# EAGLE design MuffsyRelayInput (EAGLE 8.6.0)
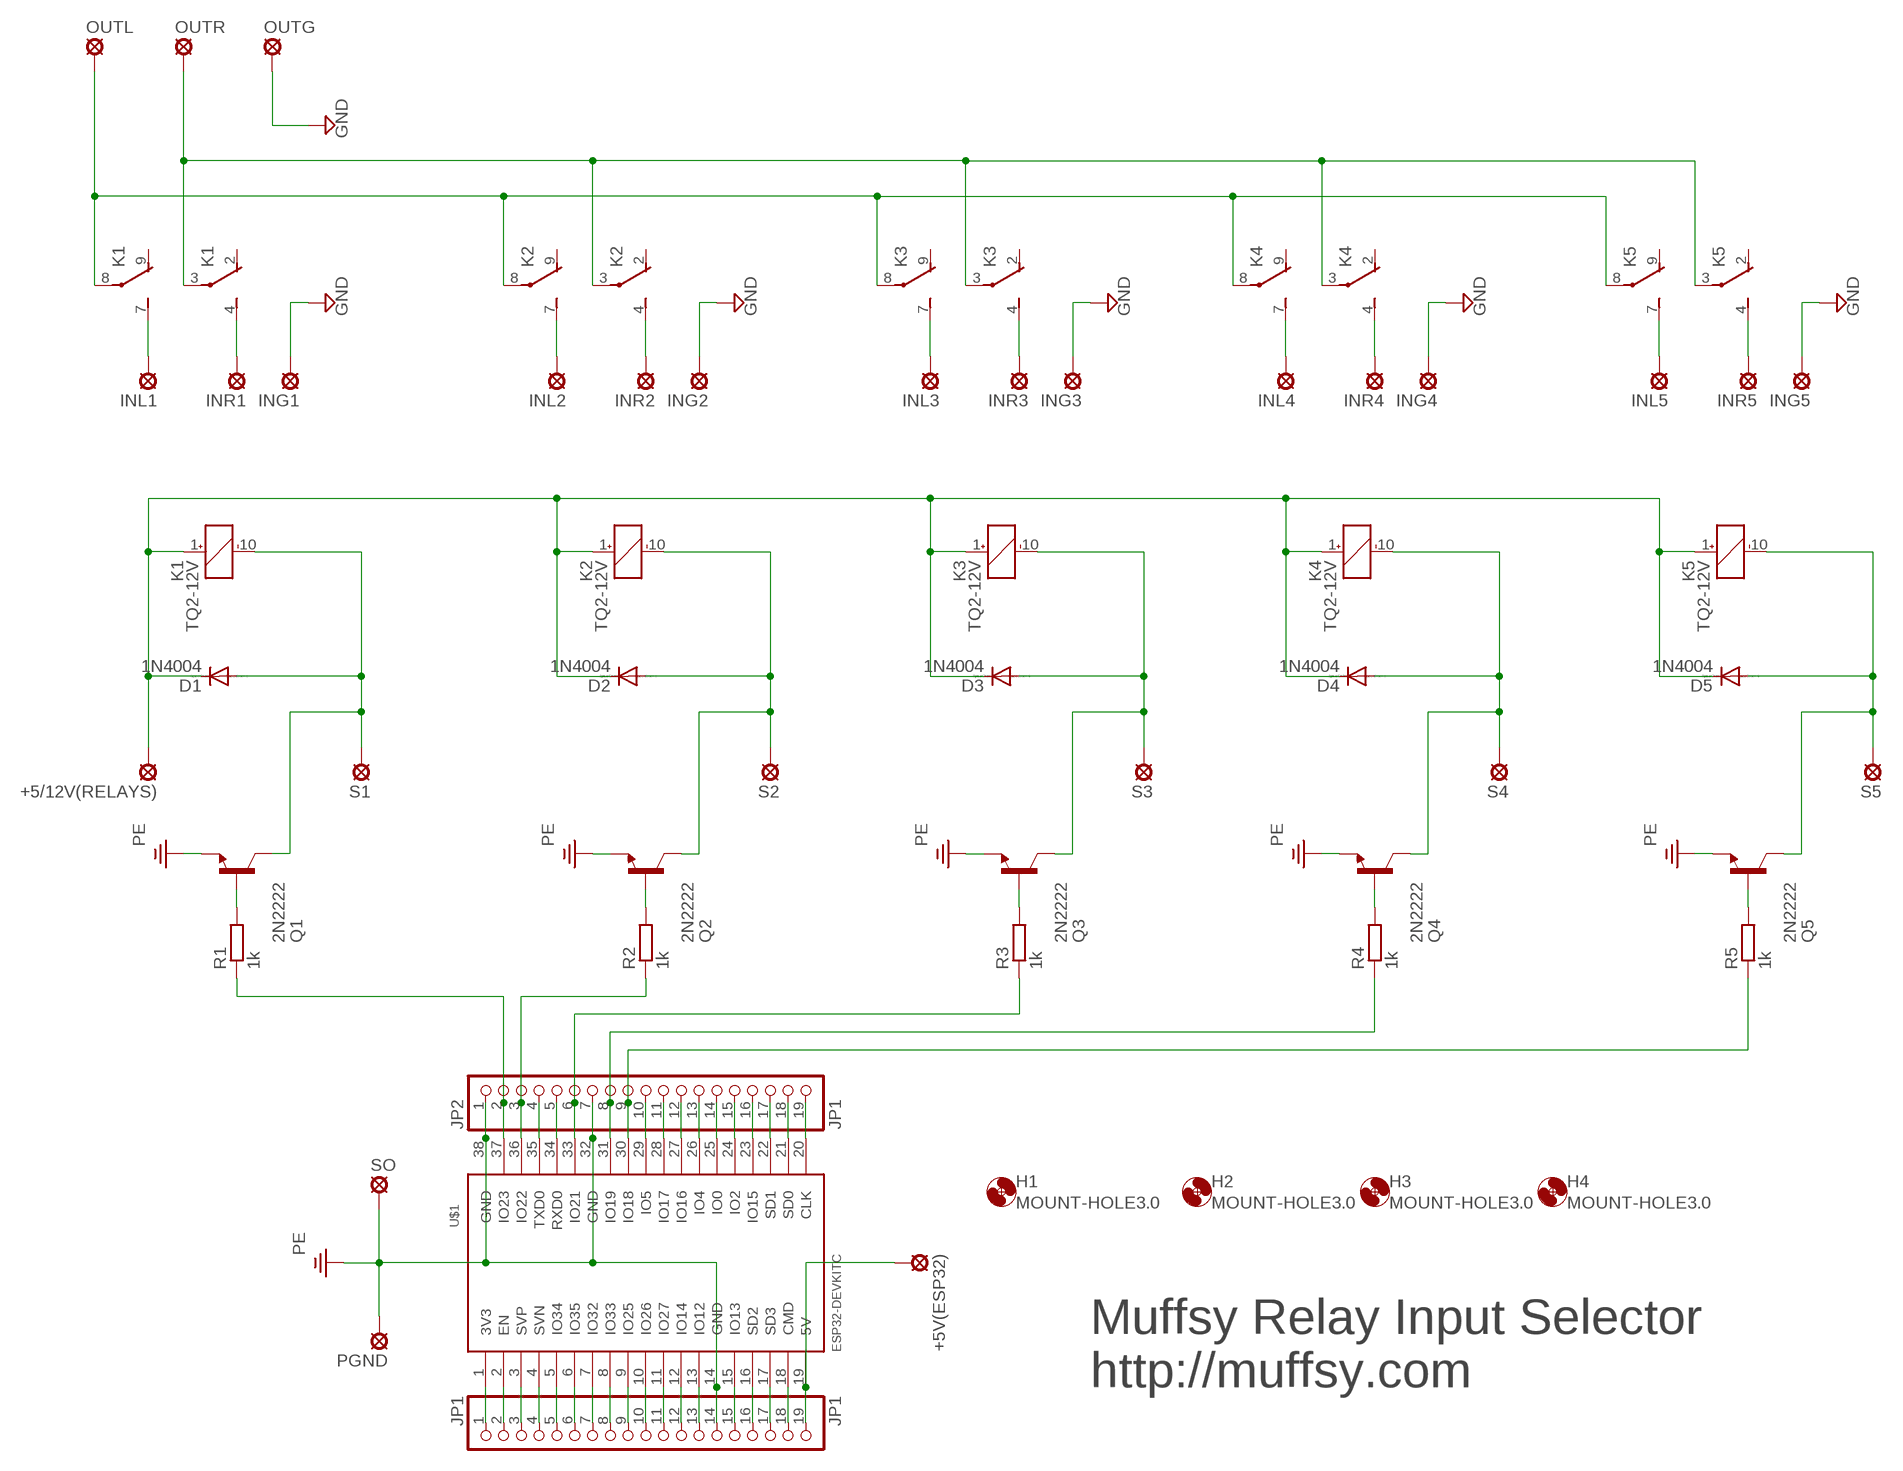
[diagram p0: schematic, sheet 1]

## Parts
+5/12V(RELAYS)  SE11  [SE11]
+5V(ESP32)  SE11  [SE11]
D1  1N4004  [DO41-10]
D2  1N4004  [DO41-10]
D3  1N4004  [DO41-10]
D4  1N4004  [DO41-10]
D5  1N4004  [DO41-10]
H1  MOUNT-HOLE3.0  [3,0]
H2  MOUNT-HOLE3.0  [3,0]
H3  MOUNT-HOLE3.0  [3,0]
H4  MOUNT-HOLE3.0  [3,0]
ING1  SE11  [SE11]
ING2  SE11  [SE11]
ING3  SE11  [SE11]
ING4  SE11  [SE11]
ING5  SE11  [SE11]
INL1  SE11  [SE11]
INL2  SE11  [SE11]
INL3  SE11  [SE11]
INL4  SE11  [SE11]
INL5  SE11  [SE11]
INR1  SE11  [SE11]
INR2  SE11  [SE11]
INR3  SE11  [SE11]
INR4  SE11  [SE11]
INR5  SE11  [SE11]
JP1  JP1  PINHD-1X19  [1X19]
JP2  JP1  PINHD-1X19  [1X19]
K1  TQ2-12V  [TQ2]
K2  TQ2-12V  [TQ2]
K3  TQ2-12V  [TQ2]
K4  TQ2-12V  [TQ2]
K5  TQ2-12V  [TQ2]
OUTG  SE11  [SE11]
OUTL  SE11  [SE11]
OUTR  SE11  [SE11]
PGND  SE11  [SE11]
Q1  2N2222  [TO18]
Q2  2N2222  [TO18]
Q3  2N2222  [TO18]
Q4  2N2222  [TO18]
Q5  2N2222  [TO18]
R1  1k  R-EU_0207/10  [0207/10]
R2  1k  R-EU_0207/10  [0207/10]
R3  1k  R-EU_0207/10  [0207/10]
R4  1k  R-EU_0207/10  [0207/10]
R5  1k  R-EU_0207/10  [0207/10]
S1  SE11  [SE11]
S2  SE11  [SE11]
S3  SE11  [SE11]
S4  SE11  [SE11]
S5  SE11  [SE11]
SO  SE11  [SE11]
U$1  ESP32DEVKITC  [ESP32-DEVKITC]

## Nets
GND: ING1.MP ING2.MP ING3.MP ING4.MP ING5.MP OUTG.MP
N$1: INL2.MP K2.7(2:S)
N$2: INL1.MP K1.7(2:S)
N$3: INR1.MP K1.4(1:S)
N$4: INR2.MP K2.4(1:S)
N$5: INL3.MP K3.7(2:S)
N$6: INR3.MP K3.4(1:S)
N$7: INL4.MP K4.7(2:S)
N$8: INR4.MP K4.4(1:S)
N$9: INL5.MP K5.7(2:S)
N$10: INR5.MP K5.4(1:S)
N$11: Q1.2(B) R1.2
N$12: K1.3(1:P) K2.3(1:P) K3.3(1:P) K4.3(1:P) K5.3(1:P) OUTR.MP
N$13: K1.8(2:P) K2.8(2:P) K3.8(2:P) K4.8(2:P) K5.8(2:P) OUTL.MP
N$14: Q2.2(B) R2.2
N$15: +5/12V(RELAYS).MP D1.C D2.C D3.C D4.C D5.C K1.1(_:+) K2.1(_:+) K3.1(_:+) K4.1(_:+) K5.1(_:+)
N$16: Q3.2(B) R3.2
N$17: Q4.2(B) R4.2
N$18: Q5.2(B) R5.2
N$19: JP1.1 U$1.1(3V3)
N$20: D1.A K1.10(_:-) Q1.3(C) S1.MP
N$21: D2.A K2.10(_:-) Q2.3(C) S2.MP
N$22: D3.A K3.10(_:-) Q3.3(C) S3.MP
N$23: D4.A K4.10(_:-) Q4.3(C) S4.MP
N$24: D5.A K5.10(_:-) Q5.3(C) S5.MP
N$25: JP1.2 U$1.2(EN)
N$26: JP1.3 U$1.3(SVP)
N$27: JP1.4 U$1.4(SVN)
N$28: JP1.5 U$1.5(IO34)
N$29: JP1.6 U$1.6(IO35)
N$30: JP1.7 U$1.7(IO32)
N$31: JP1.8 U$1.8(IO33)
N$32: JP1.9 U$1.9(IO25)
N$33: JP1.10 U$1.10(IO26)
N$34: JP1.11 U$1.11(IO27)
N$35: JP1.12 U$1.12(IO14)
N$36: JP1.13 U$1.13(IO12)
N$38: JP1.15 U$1.15(IO13)
N$44: JP1.16 U$1.16(SD2)
N$45: JP1.17 U$1.17(SD3)
N$46: JP1.18 U$1.18(CMD)
N$47: +5V(ESP32).MP JP1.19 U$1.19(5V)
N$49: JP2.2 R1.1 U$1.37(IO23)
N$50: JP2.3 R2.1 U$1.36(IO22)
N$51: JP2.4 U$1.35(TXD0)
N$52: JP2.5 U$1.34(RXD0)
N$53: JP2.6 R3.1 U$1.33(IO21)
N$55: JP2.8 R4.1 U$1.31(IO19)
N$56: JP2.9 R5.1 U$1.30(IO18)
N$57: JP2.10 U$1.29(IO5)
N$58: JP2.11 U$1.28(IO17)
N$59: JP2.12 U$1.27(IO16)
N$60: JP2.13 U$1.26(IO4)
N$61: JP2.14 U$1.25(IO0)
N$62: JP2.15 U$1.24(IO2)
N$63: JP2.16 U$1.23(IO15)
N$64: JP2.17 U$1.22(SD1)
N$65: JP2.18 U$1.21(SD0)
N$66: JP2.19 U$1.20(CLK)
PE: JP1.14 JP2.1 JP2.7 PGND.MP Q1.1(E) Q2.1(E) Q3.1(E) Q4.1(E) Q5.1(E) SO.MP U$1.14(GND) U$1.32(GND) U$1.38(GND)
Unconnected: K1.2(1:O) K1.9(2:O) K2.2(1:O) K2.9(2:O) K3.2(1:O) K3.9(2:O) K4.2(1:O) K4.9(2:O) K5.2(1:O) K5.9(2:O)

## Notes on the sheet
- Muffsy Relay Input Selector
- http://muffsy.com

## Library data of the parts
+5/12V(RELAYS) +5V(ESP32) ING1-ING5 INL1-INL5 INR1-INR5 OUTG OUTL OUTR PGND S1-S5 SO = relswitch:SE11: SOLDER PAD
D1-D5 = relswitch:1N4004: DIODE
H1-H4 = relswitch:MOUNT-HOLE: MOUNTING HOLE with drill center marker
JP1 JP2 = relswitch:PINHD-1X19: PIN HEADER
K1-K5 = relswitch:TQ2?*: LOW PROFILE 2 FORM C RELAY NAiS Source: http://www.mew-europe.com/.. en_ds_61020_0001.pdf Source: http://www.mew-europe.com/.. en_ds_61020_0004.pdf; MF: AROMAT/ MATSUSHITA; MPN: TQ2-12V; OC_FARNELL: 1200949; OC_NEWARK: 64K3197
Q1-Q5 = relswitch:2N2222*: NPN Transistor
R1-R5 = relswitch:R-EU_: RESISTOR, European symbol
U$1 = relswitch:ESP32DEVKITC

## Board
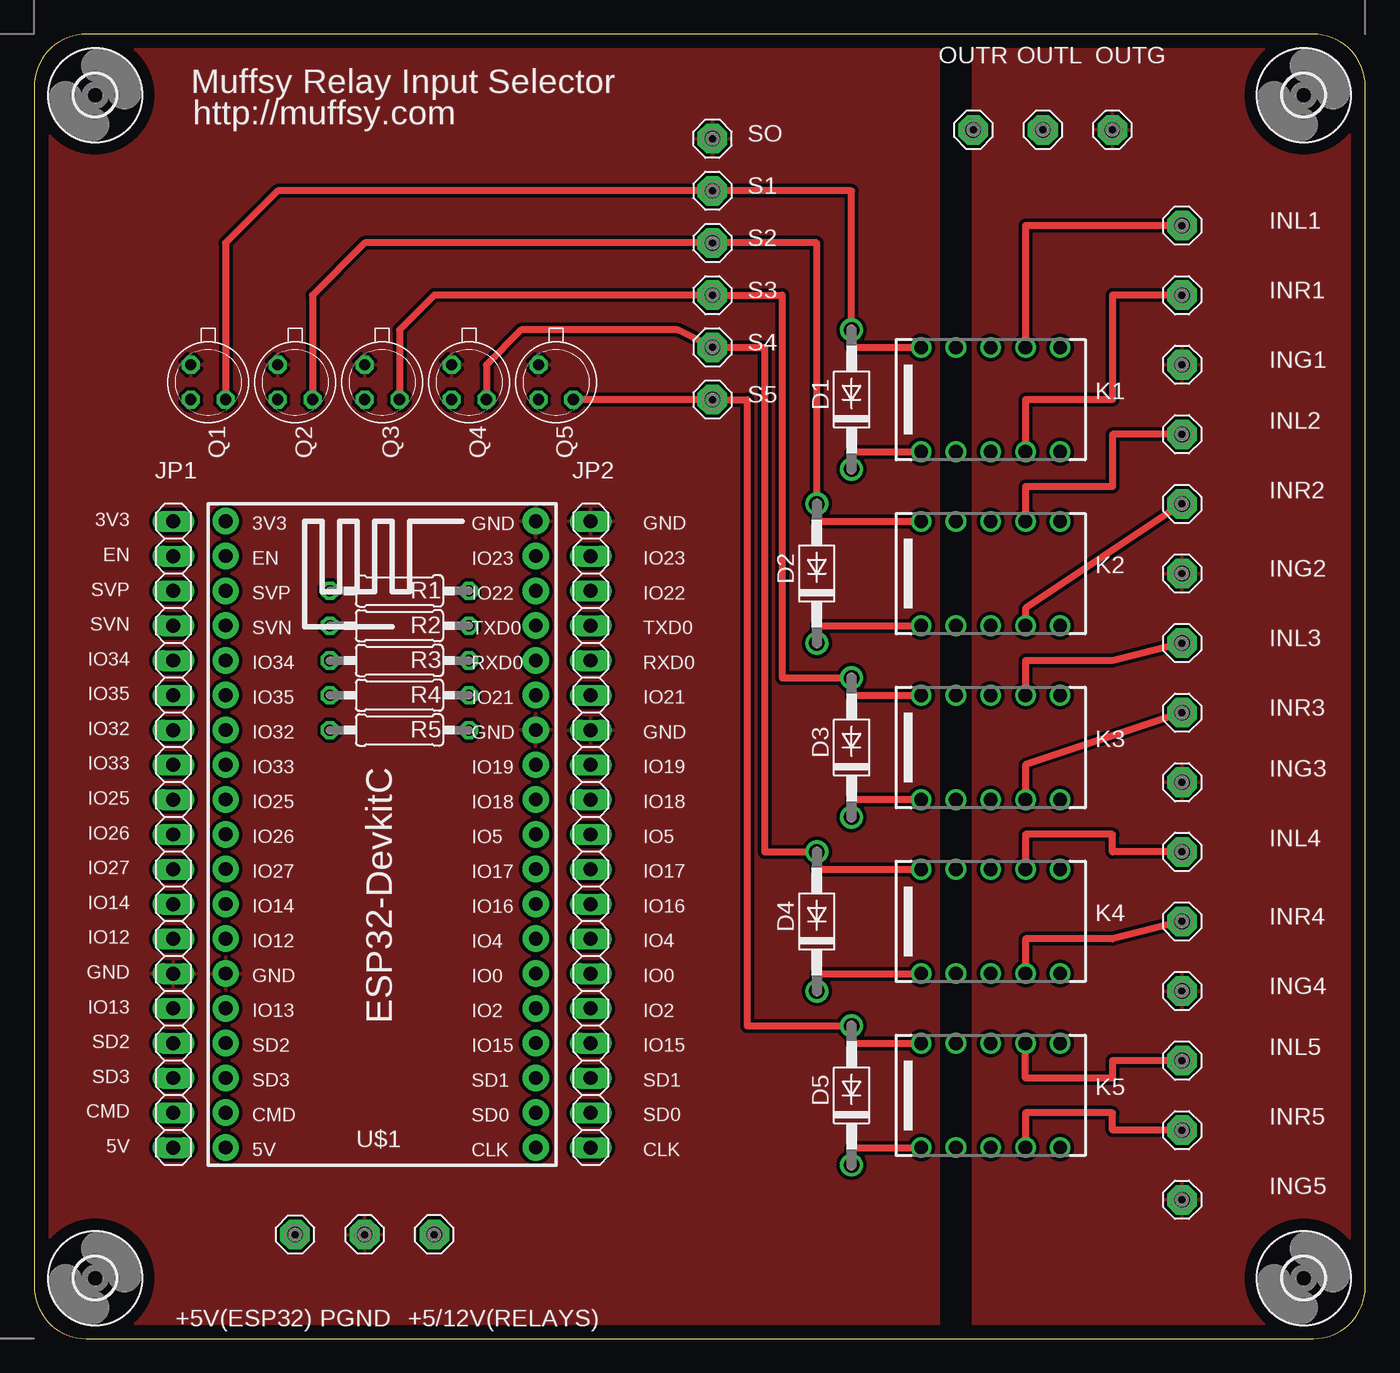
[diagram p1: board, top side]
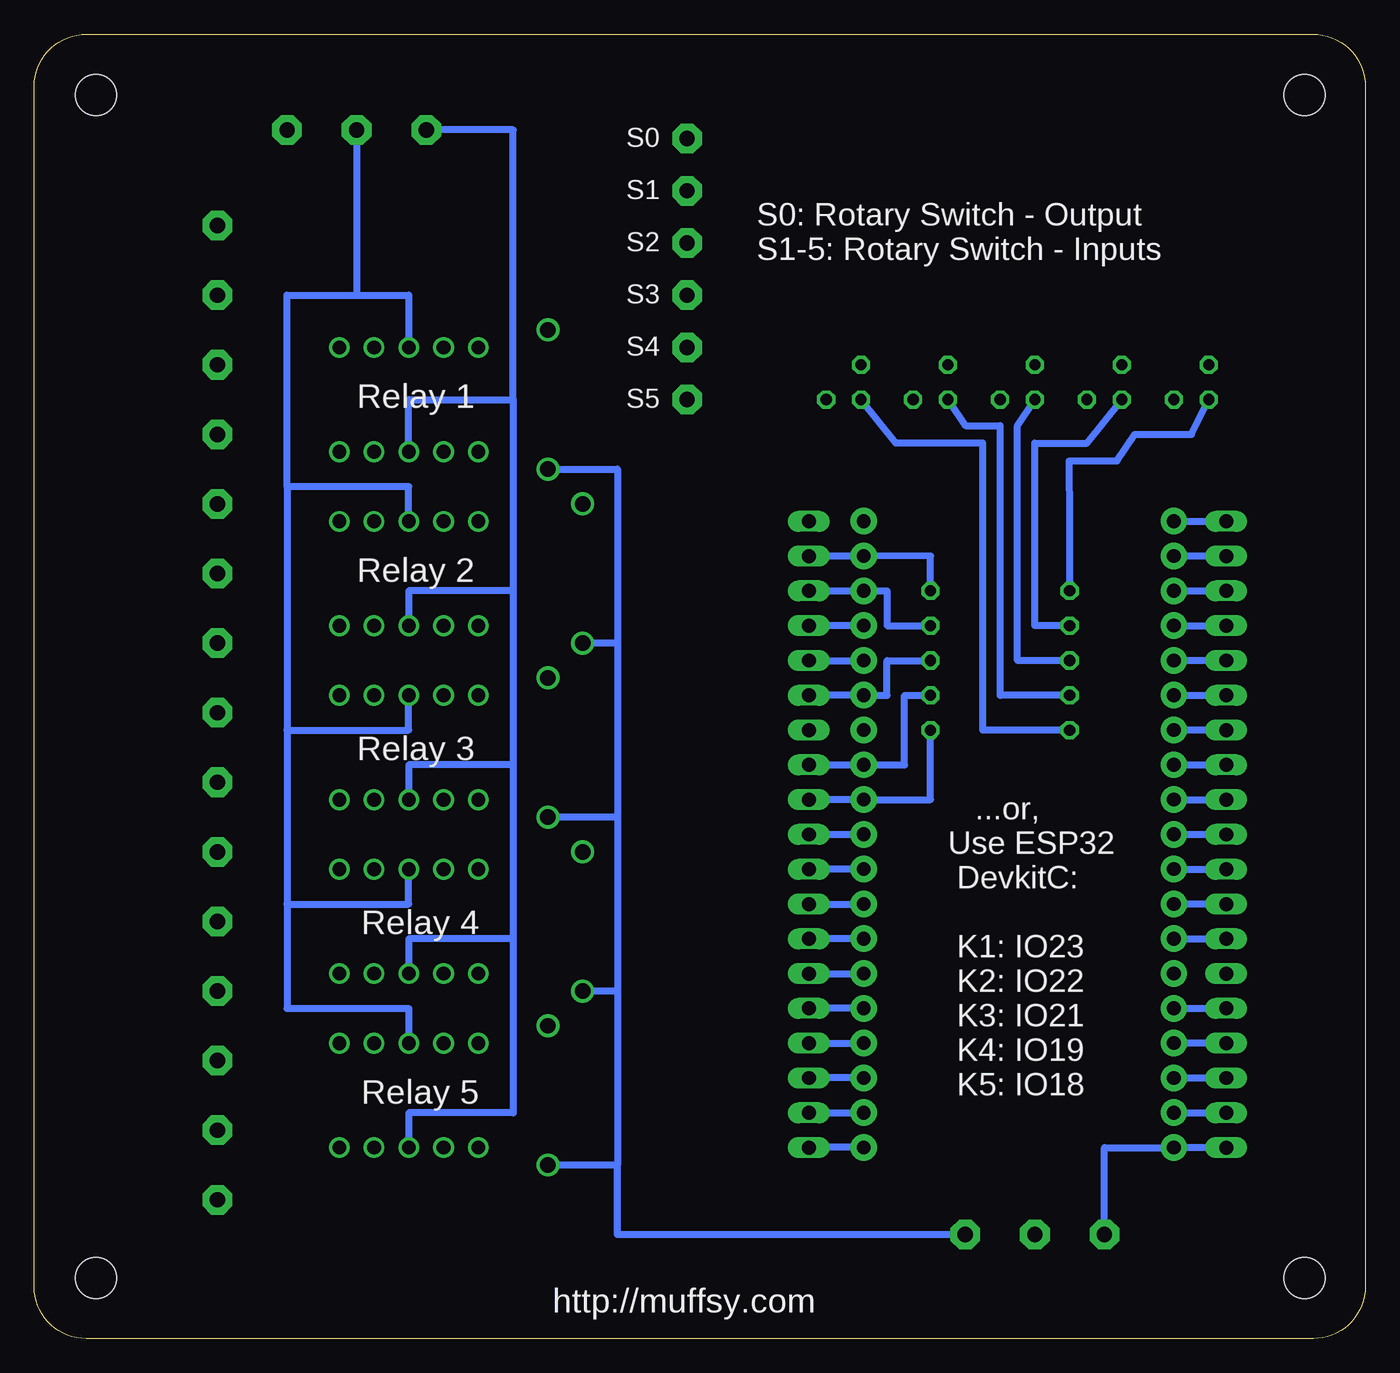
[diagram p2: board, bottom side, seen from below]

Size 97.21 x 95.23 mm. Coordinates in mm from the lower left corner, seen from the top.
Outline: 97.21,3.79 97.21,91.42 arc90 93.4,95.23 3.81,95.23 arc90 0,91.42 0,3.81 arc90 3.81,0 93.42,0 arc90 97.21,3.79
Copper layers (1*16): Top 0.035mm / dielectric 1.5mm / Bottom 0.035mm
Design rules "default": minimum track width 6mil, minimum drill 0.35mm, track to track 6mil, track to pad 6mil, pad to pad 6mil, via to via 6mil, smd to smd 6mil, copper to edge 40mil, drill to drill 6mil, minimum pad ring 10mil, minimum via ring 8mil, stop-mask expansion 4mil, vias tented up to drill 0mil, thermal gap 10mil

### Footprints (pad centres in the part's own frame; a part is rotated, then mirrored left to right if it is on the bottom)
SE11 = drill 1.118 pad 2.159 octagon: MP 0,0
DO41-10 = drill 1.118: A 5.08,0; C -5.08,0
3,0 = hole 3: 0,0
1X19 = drill 1.016 long: 1 -22.86,0; 2 -20.32,0; 3 -17.78,0; 4 -15.24,0; 5 -12.7,0; 6 -10.16,0; 7 -7.62,0; 8 -5.08,0; 9 -2.54,0; 10 0,0; 11 2.54,0; 12 5.08,0; 13 7.62,0; 14 10.16,0; 15 12.7,0; 16 15.24,0; 17 17.78,0; 18 20.32,0; 19 22.86,0
TQ2 = drill 1: 1 -5.08,-3.81; 2 -2.54,-3.81; 3 0,-3.81; 4 2.54,-3.81; 5 5.08,-3.81; 6 5.08,3.81; 7 2.54,3.81; 8 0,3.81; 9 -2.54,3.81; 10 -5.08,3.81
TO18 = drill 0.813 octagon: 1 -1.27,-1.27; 2 1.27,-1.27; 3 1.27,1.27
0207/10 = drill 0.813 octagon: 1 -5.08,0; 2 5.08,0
ESP32-DEVKITC = drill 1 pad 1.93: 1 -22.87,-11.42; 2 -20.33,-11.42; 3 -17.79,-11.42; 4 -15.25,-11.42; 5 -12.71,-11.42; 6 -10.17,-11.42; 7 -7.63,-11.42; 8 -5.09,-11.42; 9 -2.55,-11.42; 10 -0.01,-11.42; 11 2.53,-11.42; 12 5.07,-11.42; 13 7.61,-11.42; 14 10.15,-11.42; 15 12.69,-11.42; 16 15.23,-11.42; 17 17.77,-11.42; 18 20.31,-11.42; 19 22.85,-11.42; 20 22.85,11.23; 21 20.31,11.23; 22 17.77,11.23; 23 15.23,11.23; 24 12.69,11.23; 25 10.15,11.23; 26 7.61,11.23; 27 5.07,11.23; 28 2.53,11.23; 29 -0.01,11.23; 30 -2.55,11.23; 31 -5.09,11.23; 32 -7.63,11.23; 33 -10.17,11.23; 34 -12.71,11.23; 35 -15.25,11.23; 36 -17.79,11.23; 37 -20.33,11.23; 38 -22.87,11.23

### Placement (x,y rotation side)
+5/12V(RELAYS)  29.21,7.6 270 top
+5V(ESP32)  19.05,7.6 180 top
D1  59.69,68.56 90 top
D2  57.15,55.86 90 top
D3  59.69,43.16 90 top
D4  57.15,30.46 90 top
D5  59.69,17.76 90 top
H1  92.71,4.43 0 top
H2  4.45,4.43 0 top
H3  92.71,90.79 0 top
H4  4.45,90.79 0 top
ING1  83.82,71.1 0 top
ING2  83.82,55.86 0 top
ING3  83.82,40.62 0 top
ING4  83.82,25.38 0 top
ING5  83.82,10.14 0 top
INL1  83.82,81.26 0 top
INL2  83.82,66.02 0 top
INL3  83.82,50.78 0 top
INL4  83.82,35.54 0 top
INL5  83.82,20.3 0 top
INR1  83.82,76.18 0 top
INR2  83.82,60.94 0 top
INR3  83.82,45.7 0 top
INR4  83.82,30.46 0 top
INR5  83.82,15.22 0 top
JP1  10.16,36.81 270 top
JP2  40.64,36.81 270 top
K1  69.85,68.56 0 top
K2  69.85,55.86 0 top
K3  69.85,43.16 0 top
K4  69.85,30.46 0 top
K5  69.85,17.76 0 top
OUTG  78.74,88.25 270 top
OUTL  73.66,88.25 270 top
OUTR  68.58,88.25 270 top
PGND  24.13,7.6 270 top
Q1  12.7,69.83 270 top
Q2  19.05,69.83 270 top
Q3  25.4,69.83 270 top
Q4  31.75,69.83 270 top
Q5  38.1,69.83 270 top
R1  26.67,54.59 180 top
R2  26.67,52.05 180 top
R3  26.67,49.51 180 top
R4  26.67,46.97 180 top
R5  26.67,44.43 180 top
S1  49.53,83.8 0 top
S2  49.53,79.99 0 top
S3  49.53,76.18 0 top
S4  49.53,72.37 0 top
S5  49.53,68.56 0 top
SO  49.53,87.61 180 top
U$1  25.4,36.81 270 top

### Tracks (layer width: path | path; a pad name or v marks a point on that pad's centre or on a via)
GND
  pour Top (isolate 0.254): 97.16,-0.02 97.16,95.23 68.58,95.23 68.58,-0.02
N$1
  Top 0.508: K2.7 72.39,62.21 78.74,62.21 78.74,66.02 INL2.MP
N$2
  Top 0.508: INL1.MP 72.39,81.26 K1.7
N$3
  Top 0.508: INR1.MP 78.74,76.18 78.74,68.56 72.39,68.56 K1.4
N$4
  Top 0.508: INR2.MP 72.39,53.32 K2.4
N$5
  Top 0.508: INL3.MP 78.74,49.51 72.39,49.51 K3.7
N$6
  Top 0.508: INR3.MP 72.39,41.89 K3.4
N$7
  Top 0.508: K4.7 72.39,36.81 78.74,36.81 78.74,35.54 INL4.MP
N$8
  Top 0.508: INR4.MP 78.74,29.19 72.39,29.19 K4.4
N$9
  Top 0.508: INL5.MP 78.74,20.3 78.74,19.03 72.39,19.03 K5.7
N$10
  Top 0.508: INR5.MP 78.74,15.22 78.74,16.49 72.39,16.49 K5.4
N$11
  Bottom 0.508: R1.2 21.59,59.67 21.61,64.09 18.14,64.09 16.85,66.02 12.7,66.02 Q1.2
N$12
  Bottom 0.508: K1.3 69.85,68.56 62.23,68.56 | 62.23,68.56 62.23,54.59 | 62.23,54.59 69.85,54.59 K2.3 | 62.23,54.59 62.23,41.89 | 62.23,41.89 69.85,41.89 K3.3 | 62.23,41.89 62.23,29.19 | 62.23,29.19 69.85,29.19 K4.3 | 62.23,29.19 62.23,16.49 69.85,16.49 K5.3 | 62.23,68.56 62.23,88.25 OUTR.MP
N$13
  Bottom 0.508: 73.66,76.18 78.74,76.18 78.74,62.21 | 73.66,76.18 69.85,76.18 K1.8 | K2.8 69.85,62.21 78.74,62.21 | 78.74,62.21 78.74,44.43 | 78.74,44.43 69.85,44.43 K3.8 | 78.74,44.43 78.74,31.73 | 78.74,31.73 69.85,31.73 K4.8 | 78.74,31.73 78.74,24.11 69.85,24.11 K5.8 | OUTL.MP 73.66,76.18
N$14
  Bottom 0.508: R2.2 24.13,52.05 24.13,65.39 20.32,65.39 Q2.2
N$15
  Top 0.508: K1.1 59.69,64.75 D1.C | D2.C 57.15,52.05 K2.1 | D5.C 59.69,13.95 K5.1 | D4.C 57.15,26.65 K4.1 | K3.1 59.69,39.35 D3.C
  Bottom 0.508: 54.61,50.78 D2.C | 54.61,38.08 D3.C | 54.61,12.68 D5.C | 54.61,50.78 54.61,63.48 D1.C | 54.61,50.78 54.61,38.08 | 54.61,38.08 54.61,25.38 | 54.61,25.38 D4.C | 54.61,25.38 54.61,12.68 | +5/12V(RELAYS).MP 54.61,7.6 54.61,12.68
N$16
  Bottom 0.508: R3.2 25.4,49.51 25.4,66.66 Q3.2
N$17
  Bottom 0.508: R4.2 26.67,46.97 26.67,66.66 29.21,66.66 Q4.2
N$18
  Bottom 0.508: R5.2 27.94,44.43 27.94,65.39 34.29,65.39 Q5.2
N$19
  Bottom 0.508: U$1.1 JP1.1
N$20
  Top 0.508: K1.10 59.69,72.37 D1.A 59.69,83.8 S1.MP 17.78,83.8 13.97,79.99 Q1.3
N$21
  Top 0.508: K2.10 57.15,59.67 D2.A 57.15,79.99 S2.MP 24.13,79.99 20.32,76.18 Q2.3
N$22
  Top 0.508: K3.10 59.69,46.97 D3.A 54.61,48.24 54.61,76.18 S3.MP 29.21,76.18 26.67,73.64 Q3.3
N$23
  Top 0.508: K4.10 57.15,34.27 D4.A 53.34,35.54 53.34,72.37 S4.MP 46.99,73.64 35.56,73.64 33.02,71.1 Q4.3
N$24
  Top 0.508: K5.10 59.69,21.57 D5.A 52.07,22.84 52.07,68.56 S5.MP Q5.3
N$25
  Bottom 0.508: U$1.2 JP1.2
N$26
  Bottom 0.508: U$1.3 JP1.3
N$27
  Bottom 0.508: U$1.4 JP1.4
N$28
  Bottom 0.508: U$1.5 JP1.5
N$29
  Bottom 0.508: U$1.6 JP1.6
N$30
  Bottom 0.508: U$1.7 JP1.7
N$31
  Bottom 0.508: U$1.8 JP1.8
N$32
  Bottom 0.508: U$1.9 JP1.9
N$33
  Bottom 0.508: U$1.10 JP1.10
N$34
  Bottom 0.508: U$1.11 JP1.11
N$35
  Bottom 0.508: U$1.12 JP1.12
N$36
  Bottom 0.508: U$1.13 JP1.13
N$38
  Bottom 0.508: U$1.15 JP1.15
N$44
  Bottom 0.508: JP1.16 U$1.16
N$45
  Bottom 0.508: U$1.17 JP1.17
N$46
  Bottom 0.508: U$1.18 JP1.18
N$47
  Bottom 0.508: JP1.19 U$1.19 | U$1.19 | +5V(ESP32).MP 19.05,13.95 U$1.19
N$49
  Bottom 0.508: JP2.2 U$1.37 31.75,57.13 R1.1
N$50
  Bottom 0.508: JP2.3 36.83,54.59 36.82,54.6 U$1.36 34.92,54.59 34.92,52.05 R2.1
N$51
  Bottom 0.508: U$1.35 JP2.4
N$52
  Bottom 0.508: U$1.34 JP2.5
N$53
  Bottom 0.508: JP2.6 U$1.33 34.92,46.97 34.92,49.51 R3.1
N$55
  Bottom 0.508: JP2.8 U$1.31 33.66,41.89 33.66,46.97 R4.1
N$56
  Bottom 0.508: JP2.9 U$1.30 31.75,39.35 R5.1
N$57
  Bottom 0.508: JP2.10 36.83,36.81 36.82,36.82 U$1.29
N$58
  Bottom 0.508: U$1.28 JP2.11
N$59
  Bottom 0.508: JP2.12 U$1.27
N$60
  Bottom 0.508: U$1.26 JP2.13
N$61
  Bottom 0.508: JP2.14 U$1.25
N$62
  Bottom 0.508: U$1.24 JP2.15
N$63
  Bottom 0.508: JP2.16 36.83,21.57 36.82,21.58 U$1.23
N$64
  Bottom 0.508: U$1.22 JP2.17
N$65
  Bottom 0.508: JP2.18 U$1.21
N$66
  Bottom 0.508: U$1.20 JP2.19
PE
  pour Top (isolate 0.254, rank 5): 0,95.23 0,-0.02 66.04,-0.02 66.04,95.23

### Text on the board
tNames: Muffsy Relay Input Selector | http://muffsy.com | 3V3 / EN / SVP / SVN / IO34 / IO35 / IO32 / IO33 / IO25 / IO26 / IO27 / IO14 / IO12 / GND / IO13 / SD2 / SD3 / CMD / 5V | GND / IO23 / IO22 / TXD0 / RXD0 / IO21 / GND / IO19 / IO18 / IO5 / IO17 / IO16 / IO4 / IO0 / IO2 / IO15 / SD1 / SD0 / CLK
bNames: S0 | S1 | S0: Rotary Switch - Output / S1-5: Rotary Switch - Inputs | S2 | S3 | S4 | S5 | Relay 1 | Relay 2 | Relay 3 | Relay 4 | ...or, / Use ESP32 / DevkitC: / / K1: IO23 / K2: IO22 / K3: IO21 / K4: IO19 / K5: IO18 | Relay 5 | http://muffsy.com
